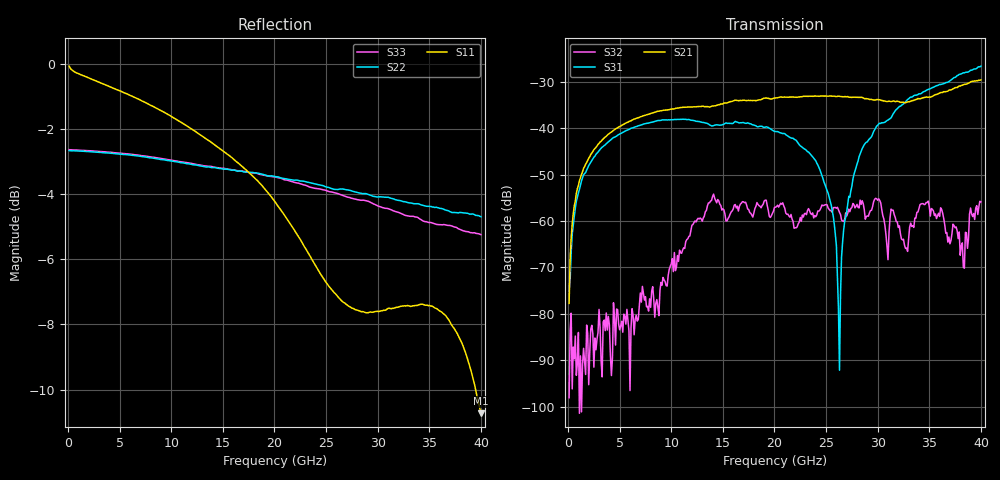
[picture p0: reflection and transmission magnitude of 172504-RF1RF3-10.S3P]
!  3-Port S-parameters saved by WinCal
! VAR MeasName=S-Parameters (CALIBRATED_DATA) read from VNA (N5245A)
! VAR MeasDate=2017-3-15 11:05:36
! VAR NAME=172504-RF1RF3-10
! VAR FILENAME=172504-RF1RF3-10.S3P
! VAR DATE=2017-3-15 11:05:36
! VAR PHYS_PORTS=1,2,3
# Hz S DB R 50
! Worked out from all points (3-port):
!   400 points, 100 MHz to 40 GHz, reference 50 ohm
!   strongest paths, dB at 100 MHz, 10.1 GHz, 20.1 GHz, 30.1 GHz, 40 GHz:
!     S21: -77.8, -35.8, -33.5, -33.9, -29.6
!     S31: -75.1, -38.2, -40.7, -39.1, -26.6
!     S32: -98.1, -68.1, -57.0, -55.2, -55.9
!   lowest |S11| = -10.7 dB at 40 GHz (marker M1), VSWR 1.82, Z = 29.5 - j11.1 ohm
!   |S11| at or under -10 dB: 39.49 GHz to end of sweep
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1e8  -0.07 -2.0  -75.28 123.7  -80.86 166.3
     -77.75 91.2  -2.66 179.8  -80.67 9.0
     -75.08 87.5  -98.10 28.1  -2.63 179.8
8e8  -0.27 -12.3  -54.20 90.6  -55.66 95.3
     -53.98 90.0  -2.67 178.3  -98.93 -79.7
     -55.79 93.6  -93.27 61.0  -2.64 178.3
3.4e9  -0.61 -48.1  -42.30 63.1  -43.91 56.0
       -42.31 63.1  -2.73 172.8  -83.03 85.4
       -43.94 56.3  -81.76 49.9  -2.70 173.0
1.19e10  -1.98 -140.3  -35.44 12.5  -38.25 -21.5
         -35.45 12.4  -3.08 155.5  -62.31 173.6
         -38.28 -21.6  -62.01 168.2  -3.05 156.1
2.01e10  -4.26 139.4  -33.46 -18.0  -40.63 -76.8
         -33.48 -17.2  -3.46 137.8  -56.94 72.2
         -40.71 -76.6  -57.02 68.6  -3.47 138.5
2.52e10  -6.80 66.2  -33.01 -42.3  -53.75 -127.0
         -33.09 -41.0  -3.79 125.5  -56.95 58.7
         -54.01 -125.5  -57.22 56.2  -3.91 125.9
2.63e10  -7.21 47.2  -32.99 -47.6  -91.20 -61.7
         -33.12 -46.8  -3.84 123.1  -57.89 50.6
         -92.18 15.2  -58.15 46.8  -4.00 123.1
2.86e10  -7.61 7.7  -33.34 -59.6  -43.53 27.9
         -33.46 -57.8  -3.98 116.9  -56.75 39.4
         -43.94 28.5  -56.27 42.2  -4.18 117.0
3.84e10  -8.78 -120.1  -30.22 -80.8  -27.78 -86.7
         -30.55 -77.3  -4.58 88.2  -70.27 131.8
         -28.06 -83.0  -70.18 111.1  -5.13 87.7
4e10  -10.73 -143.7  -29.24 -90.8  -26.47 -104.9
      -29.58 -86.8  -4.69 82.6  -55.40 132.5
      -26.63 -99.5  -55.87 136.7  -5.24 82.5
